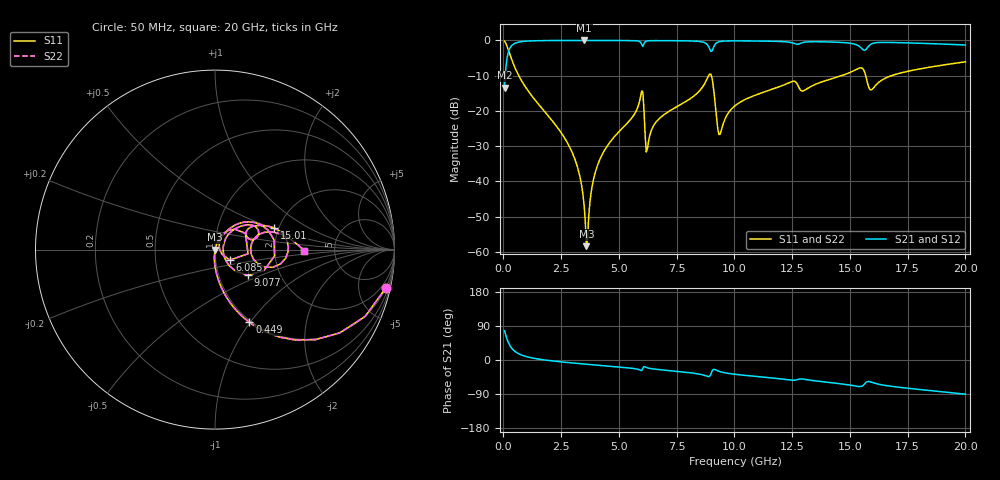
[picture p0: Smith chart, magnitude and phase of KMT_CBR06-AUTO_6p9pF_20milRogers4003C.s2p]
! Data measured by Modelithics Inc. support@modelithics.com 813-866-6335
! KEMET CBR06-AUTO 6.9pF, Pad Width= 0.851mm, Pad Length= 0.64mm, Pad Gap= 0.62mm, 20mil Rogers 4003C substrate Data, January 2022
# hz S ma R 50
! 2 Port Network Data from SP1.SP block
! freq  magS11  angS11  magS21  angS21  magS12  angS12  magS22  angS22
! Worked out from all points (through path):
!   401 points, 50 MHz to 20 GHz, reference 50 ohm
!   highest |S21| = -0.01 dB at 3.491 GHz (marker M1); lowest = -13.4 dB at 50 MHz (marker M2)
!   group delay of S21, straight-line fit = 13.9 ps
!   lowest |S11| = -58.4 dB at 3.591 GHz (marker M3), VSWR 1.00, Z = 50.1 - j0.0889 ohm
!   |S11| at or under -10 dB: 663.7 MHz to 8.882 GHz (8.218 GHz wide, 172 % of centre); 9 GHz to 14.63 GHz (5.634 GHz wide, 47.7 % of centre); 15.68 GHz to 16.8 GHz (1.114 GHz wide, 6.86 % of centre)
!   |S22| runs from -58.4 to -0.2 dB; largest |S21 - S12| = 0
!   S11 on the Smith chart (normalised r, x): 50 MHz: 0.98, -9.03; 449 MHz: 0.98, -0.99; 6.085 GHz: 1.17, -0.14; 9.077 GHz: 1.38, -0.41; 15.01 GHz: 1.90, +0.52; 20 GHz: 2.98, -0.06
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5e7  0.9768 -12.5  0.2138 77.5  0.2138 77.5  0.9768 -12.5
4.49e8  0.4481 -64.7  0.8934 25.2  0.8934 25.2  0.4481 -64.7
2.793125e9  0.03414 -95.3  0.9985 -6.7  0.9985 -6.7  0.03414 -95.3
3.391625e9  0.008457 -93.7  0.9989 -10.1  0.9989 -10.1  0.008457 -93.7
3.491375e9  0.004619 -88.6  0.9989 -10.6  0.9989 -10.6  0.004619 -88.6
3.591125e9  0.001208 -47.3  0.9989 -11.1  0.9989 -11.1  0.001208 -47.3
3.94025e9  0.01217 72.2  0.9987 -13.0  0.9987 -13.0  0.01217 72.2
4.289375e9  0.02457 72.6  0.9984 -14.8  0.9984 -14.8  0.02457 72.6
5.93525e9  0.1583 46.0  0.9423 -27.1  0.9423 -27.1  0.1583 46.0
6.084875e9  0.1015 -35.2  0.9028 -17.1  0.9028 -17.1  0.1015 -35.2
6.2345e9  0.02947 38.0  0.9842 -20.8  0.9842 -20.8  0.02947 38.0
6.73325e9  0.07717 62.4  0.9936 -25.3  0.9936 -25.3  0.07717 62.4
8.72825e9  0.2494 38.3  0.9233 -41.2  0.9233 -41.2  0.2494 38.3
9.077375e9  0.2333 -37.3  0.7704 -25.2  0.7704 -25.2  0.2333 -37.3
9.376625e9  0.04657 11.4  0.9647 -30.7  0.9647 -30.7  0.04657 11.4
1.0025e10  0.1184 48.6  0.9849 -37.7  0.9849 -37.7  0.1184 48.6
1.336662e10  0.2276 32.2  0.9586 -54.0  0.9586 -54.0  0.2276 32.2
1.50125e10  0.3523 19.8  0.9121 -66.4  0.9121 -66.4  0.3523 19.8
1.551125e10  0.407 -1.9  0.7698 -69.3  0.7698 -69.3  0.407 -1.9
1.591025e10  0.1986 0.7  0.8823 -58.2  0.8823 -58.2  0.1986 0.7
1.670825e10  0.3085 18.6  0.9363 -68.7  0.9363 -68.7  0.3085 18.6
2e10  0.4972 -0.9  0.8611 -90.2  0.8611 -90.2  0.4972 -0.9
